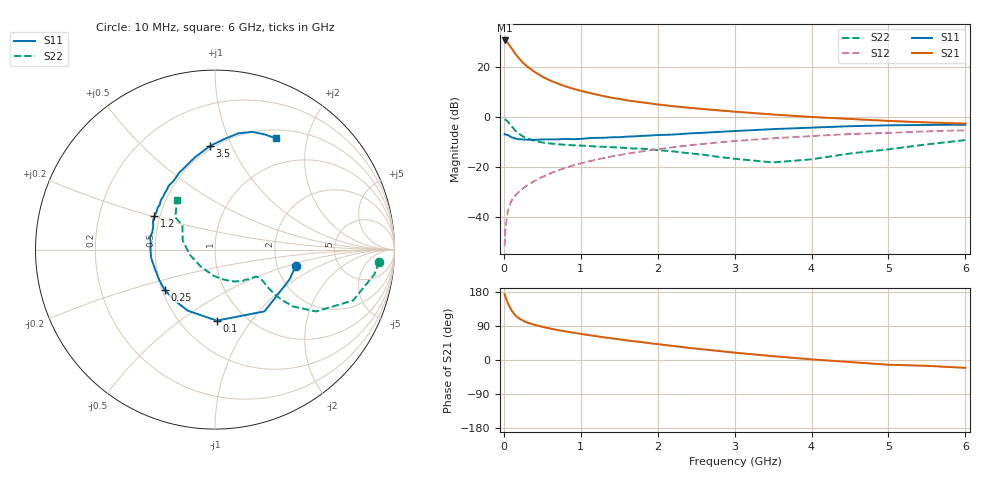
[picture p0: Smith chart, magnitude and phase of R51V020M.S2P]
! SIEMENS Small Signal Semiconductors
! BFR183
! Si NPN RF Bipolar Junction Transistor in SOT23
! VCE = 1 V  IC = 20 mA
! Common Emitter S-Parameters:  May  1996
# GHz  S  MA  R  50
!  f  S11  S21  S12  S22
! GHz  MAG  ANG  MAG  ANG  MAG  ANG  MAG  ANG
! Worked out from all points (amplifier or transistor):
!   36 points, 10 MHz to 6 GHz, reference 50 ohm
!   highest |S21| = 30.8 dB at 10 MHz (marker M1)
!   |S21| within 3 dB of that: start of sweep to 96.67 MHz
!   unconditionally stable (mu >= 1): 390.8 MHz to 2.806 GHz
!   at 250 MHz: K = 0.87, MSG = 25.1 dB, |S12| = -28.5 dB
!   at 1.4 GHz: K = 1.09, MAG = 10.0 dB, |S12| = -15.7 dB
!   at 6 GHz: K = 0.96, MSG = 1.3 dB, |S12| = -5.2 dB
!   S11 on the Smith chart (normalised r, x): 10 MHz: 2.54, -0.58; 100 MHz: 0.74, -0.70; 250 MHz: 0.52, -0.26; 1.2 GHz: 0.47, +0.20; 3.5 GHz: 0.48, +0.83; 6 GHz: 0.61, +1.51
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0.01  0.459 -11.3  34.55 173.6  0.0026 83.1  0.9165 -4.3
0.02  0.4476 -21.8  34.12 167.2  0.0056 78.8  0.8987 -8.8
0.05  0.441 -51.3  30.97 150.7  0.0128 72.5  0.8203 -20.2
0.1  0.3958 -88.5  24.05 130.8  0.0214 65.9  0.6597 -31.5
0.15  0.3727 -113.9  18.59 117.6  0.0269 62.9  0.5373 -36.1
0.2  0.3618 -129.4  14.97 109.6  0.0324 63.4  0.463 -37.0
0.25  0.3587 -141.5  12.3 103.7  0.0376 64.9  0.4104 -36.7
0.3  0.3541 -151.1  10.47 99.2  0.0426 65.9  0.3762 -36.0
0.4  0.3519 -163.0  8.078 92.9  0.0528 67.5  0.3358 -34.2
0.5  0.3585 -172.4  6.523 87.5  0.0635 68.4  0.3119 -32.9
0.6  0.3595 -179.5  5.47 83.1  0.0744 68.9  0.2978 -32.5
0.7  0.3597 173.9  4.727 79.0  0.0854 69.0  0.288 -32.5
0.8  0.3681 169.8  4.155 75.4  0.0964 68.5  0.2794 -32.9
1.1  0.3796 155.7  3.1 65.9  0.1296 66.7  0.265 -36.0
1.2  0.3859 151.3  2.858 62.8  0.1409 65.8  0.2583 -37.2
1.6  0.4087 137.5  2.184 51.7  0.1852 61.5  0.2395 -44.5
2.2  0.4484 120.5  1.661 37.1  0.2503 54.4  0.207 -59.1
2.8  0.5085 105.7  1.369 23.7  0.3132 46.3  0.1594 -81.4
3.5  0.5773 92.9  1.132 10.1  0.3778 36.1  0.1238 -129.1
4.5  0.6605 78.7  0.923 -5.4  0.4597 22.4  0.1873 164.1
5.5  0.6993 66.5  0.785 -15.4  0.5209 10.4  0.2855 141.0
6  0.7059 61.4  0.745 -20.7  0.5476 2.8  0.347 127.4
